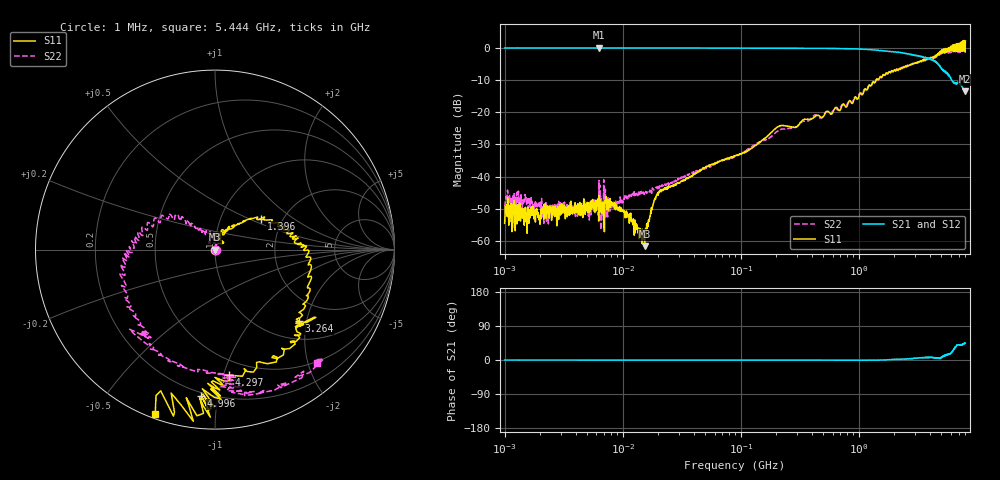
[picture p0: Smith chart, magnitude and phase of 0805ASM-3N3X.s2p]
!s-Parameter Generated by FASTRON Sdn. Bhd.
!FASTRON P/N : 0805ASM-3N3X
!Keysight Technologies: E5071C_MY46733604_B.14.02
!Date: Fri Jun 19 14:46:15 2026
!Version  :Rev00  Fri Jun 19 14:46:15 2026
!Data & Calibration Information:
!Freq  S11:SOLT2(ON)  S21:SOLT2(ON)  S12:SOLT2(ON)  S22:SOLT2(ON)
!PortZ  Port1:50+j0  Port2:50+j0
!When reading reference impedance value at option line is always used.
! Remarks : This data is being provided solely for informational purposes.
# Hz S dB R 50
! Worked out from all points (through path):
!   1601 points, 1 MHz to 8 GHz, reference 50 ohm
!   highest |S21| = 0.02 dB at 6.301 MHz (marker M1); lowest = -13.5 dB at 7.923 GHz (marker M2)
!   lowest |S11| = -61.6 dB at 15.35 MHz (marker M3), VSWR 1.00, Z = 50.1 + j0.0348 ohm
!   |S11| at or under -10 dB: start of sweep to 1.403 GHz
!   |S22| runs from -56.5 to -0.2 dB; largest |S21 - S12| = 0.0089
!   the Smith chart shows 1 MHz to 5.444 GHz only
!   S11 on the Smith chart (normalised r, x): 1 MHz: 1.00, -0.00; 1.396 GHz: 1.55, +0.59; 3.264 GHz: 1.41, -1.79; 4.297 GHz: 0.38, -1.05; 4.996 GHz: 0.18, -0.90; 5.444 GHz: 0.02, -0.70
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1000000  -54.50 -33.4  -0.04 -0.1  -0.03 -0.1  -48.80 -4.1
2361828  -50.90 12.7  -0.04 -0.0  -0.03 -0.0  -52.50 31.4
4479405  -50.20 6.3  -0.04 -0.0  -0.04 -0.1  -50.80 15.3
6301378  -45.70 21.2  0.02 -0.2  -0.01 -0.2  -41.20 34.7
9831976  -50.10 19.2  -0.03 -0.1  -0.04 -0.1  -46.90 27.3
1.535471e7  -61.60 24.7  -0.03 -0.1  -0.05 -0.1  -44.60 31.0
2.00676e7  -45.00 44.7  -0.04 -0.1  -0.05 -0.1  -43.40 54.7
8.994653e7  -33.50 74.7  -0.06 -0.3  -0.07 -0.3  -33.70 72.8
2.111884e8  -24.40 38.2  -0.10 -0.2  -0.11 -0.3  -25.60 130.0
4.006501e8  -22.00 94.8  -0.14 -0.2  -0.15 -0.2  -21.60 80.8
1.395953e9  -10.20 34.1  -0.75 -0.6  -0.76 -0.8  -10.00 142.0
1.7949e9  -7.53 15.3  -1.17 0.9  -1.18 0.6  -7.43 163.0
2.486897e9  -5.69 -0.3  -1.78 3.1  -1.84 2.8  -5.67 -175.0
3.26428e9  -4.26 -40.4  -2.64 6.2  -2.65 6.4  -4.32 -132.0
3.730463e9  -3.73 -47.1  -3.21 6.0  -3.21 6.2  -3.65 -122.0
4.296652e9  -3.05 -83.6  -3.89 5.3  -3.88 4.9  -3.15 -85.7
4.996448e9  -1.71 -95.3  -6.45 5.5  -6.47 5.4  -1.72 -74.6
5.444317e9  -0.23 -110.0  -7.30 13.2  -7.34 12.8  -1.41 -47.9
6.457806e9  -0.14 -123.0  -11.00 28.7  -10.90 28.5  -0.69 5.0
6.959019e9  -0.75 -142.0  -11.00 39.7  -11.00 39.0  -0.95 45.8
7.92289e9  1.44 -162.0  -13.50 44.4  -13.20 43.9  -0.20 78.5
8e9  2.14 -176.0  -13.30 44.4  -13.20 44.1  -0.34 75.9
